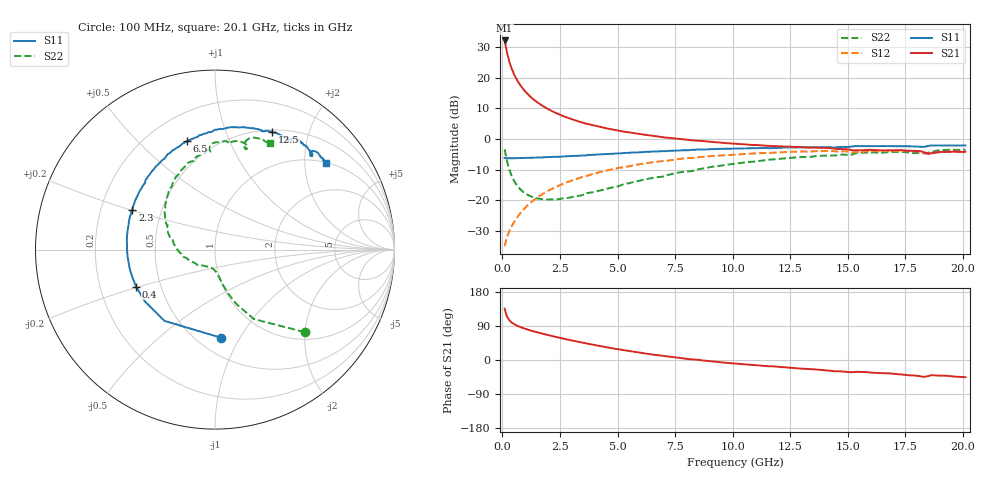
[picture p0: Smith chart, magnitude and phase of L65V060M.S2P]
!  Infineon Technologies AG
! BFR380L3 , PF131585-7, No.6, Th 09.10.01, soldered on pcb-board, measured with PP GSG850
!  Vce=5.0 V,  Ic=60.0 mA
! Common Emitter S-Parameters:  15. November 2001
#  GHz  S  MA  R  50
! f  S11  S21  S12  S22
! GHz  Mag  Ang  Mag  Ang  Mag  Ang  Mag  Ang
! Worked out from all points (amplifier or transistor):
!   201 points, 100 MHz to 20.1 GHz, reference 50 ohm
!   highest |S21| = 32.2 dB at 100 MHz (marker M1)
!   |S21| within 3 dB of that: start of sweep to 177.8 MHz
!   unconditionally stable (mu >= 1): 865.4 MHz to 4.249 GHz; 18.32 GHz to 18.53 GHz
!   at 3.4 GHz: K = 1.02, MAG = 8.1 dB, |S12| = -12.6 dB
!   at 10.1 GHz: K = 0.95, MSG = 1.8 dB, |S12| = -5.1 dB
!   at 20.1 GHz: K = 0.99, MSG = 0.0 dB, |S12| = -4.0 dB
!   S11 on the Smith chart (normalised r, x): 100 MHz: 0.64, -0.83; 400 MHz: 0.36, -0.20; 2.3 GHz: 0.34, +0.20; 6.5 GHz: 0.36, +0.71; 12.5 GHz: 0.52, +1.46; 20.1 GHz: 1.01, +2.54
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0.1  0.4913 -86.3  40.92 135.4  0.01774 61.2  0.6804 -42.6
0.2  0.4867 -125.3  26.25 115.1  0.02471 57.6  0.4429 -60.8
0.3  0.4857 -143.6  18.71 105.4  0.03091 59.1  0.3217 -68.9
0.4  0.4856 -154.8  14.4 99.4  0.03705 61.7  0.2533 -73.5
0.5  0.4856 -161.6  11.66 95.0  0.04326 63.7  0.2111 -76.5
0.6  0.4868 -167.3  9.792 91.8  0.04966 65.5  0.1828 -78.8
0.7  0.4864 -171.7  8.442 88.9  0.05584 66.7  0.1627 -80.8
0.8  0.4885 -175.2  7.415 86.5  0.06262 67.7  0.1482 -82.6
1  0.4904 178.8  5.974 82.2  0.07578 68.7  0.1287 -85.9
1.2  0.4938 174.0  5.004 78.4  0.08927 68.9  0.1173 -89.6
1.5  0.4978 167.9  4.039 73.3  0.1094 68.7  0.1076 -95.2
1.8  0.5032 162.6  3.391 68.6  0.1296 67.7  0.1033 -101.4
2.3  0.5112 154.2  2.698 61.2  0.163 65.5  0.1032 -112.5
3.5  0.5375 137.2  1.846 45.3  0.2418 58.4  0.1226 -136.0
4.9  0.5787 120.7  1.407 29.6  0.3278 49.2  0.1651 -163.1
6.5  0.6238 104.3  1.134 14.5  0.4163 38.1  0.2304 172.5
6.8  0.63 101.5  1.094 12.1  0.431 35.8  0.24 168.2
10.1  0.7 76.8  0.8373 -9.3  0.5588 13.6  0.3963 132.4
12.5  0.7303 64.3  0.7496 -20.3  0.6185 -1.7  0.4915 110.0
13.5  0.7349 59.4  0.7265 -24.6  0.6296 -7.8  0.5193 102.6
16.8  0.7641 47.1  0.6574 -35.2  0.6356 -24.2  0.6126 80.0
20.1  0.7843 38.2  0.6204 -45.2  0.6275 -38.2  0.6696 62.9
